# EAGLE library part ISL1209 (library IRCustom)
ISL1209 Low Power RTC with Battery Backed SRAM and Event Detection The ISL1209 device is a low power real time clock with event detect function, timing and crystal compensation, clock/calendar, power fail indicator, periodic or polled alarm, intelligent battery backup switching and battery-backed user SRAM.
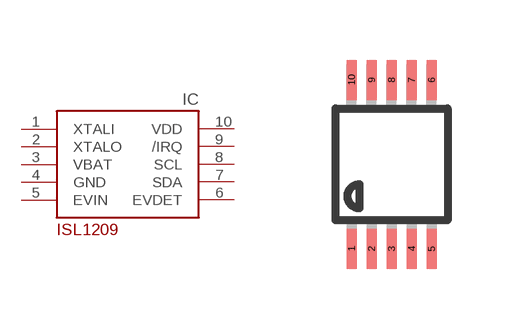
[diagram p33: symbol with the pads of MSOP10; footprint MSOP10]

Designator prefix IC

## ISL1209  [MSOP10]
1  XTALI  in
2  XTALO  out
3  VBAT  pwr
4  GND  pwr
5  EVIN  in
6  EVDET  out
7  SDA
8  SCL  in
9  /IRQ  out
10  VDD  pwr

## Footprint MSOP10 (pad centres in mm)
10-Lead Mini Small Outline Package [MSOP]
smd 0.25 x 1: 1 -1,-2.113; 2 -0.5,-2.113; 3 0,-2.113; 4 0.5,-2.113; 5 1,-2.113; 6 1,2.113; 7 0.5,2.113; 8 0,2.113; 9 -0.5,2.113; 10 -1,2.113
